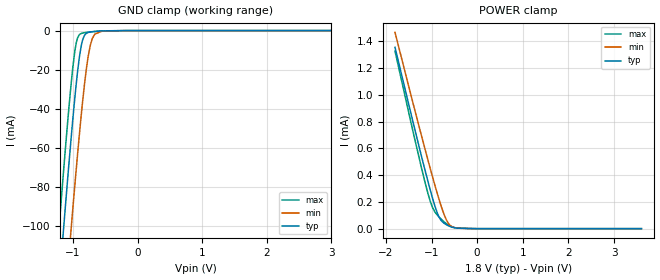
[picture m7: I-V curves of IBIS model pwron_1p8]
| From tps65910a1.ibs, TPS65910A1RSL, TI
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|   pwron_1p8 Model
[Model]   pwron_1p8
Model_type   Input
Vinl = 0.54
Vinh = 1.26
|   typ   min   max
|   (nom PVT)   (fast PVT)   (slow PVT)
C_comp   1.767e-13   1.755e-13   1.788e-13
[Model spec]
|subparameter
Vinl   0.54   0.495   0.585
Vinh   1.26   1.155   1.365
| Where nom  PVT is Nominal Process, 1.8V, 27C
|   Fast PVT is Strong Process,  1.95V, -40C
|   Slow PVT is Weak Process,   1.65V, 125C
[Voltage Range]   1.8   1.65   1.95
|Junction Temperature
[Temperature Range]   27   125   -40
[Power Clamp Reference]   1.8   1.65   1.95
[GND Clamp Reference]   0   0   0
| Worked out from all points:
|   GND clamp passes 1 mA (typ) near -0.77 V on its own axis
[GND Clamp]
|   Voltage   I(typ)   I(min)   I(max)
-1.8V     -386.3mA   -432.6mA   -358.2mA
-1.404V   -211.1mA   -258.7mA   -181.7mA
-1.205V   -125.8mA   -173.7mA   -96.01mA
-1.168V   -110.4mA   -158.2mA   -80.59mA
-1.123V   -91.91mA   -139.6mA   -62.35mA
-1.018V   -50.62mA   -96.93mA   -23.29mA
-948.6mV  -26.62mA   -70.23mA   -6.002mA
-876.6mV  -8.368mA   -44.47mA   -1.52mA
-803.4mV  -1.665mA   -22.12mA   -996.5uA
-733.3mV  -734.1uA   -7.619mA   -701.3uA
-551mV    -175.5uA   -315.4uA   -135.6uA
3.6V      0A         0A         0A
[POWER Clamp]
|   Voltage   I(typ)   I(min)   I(max)
-1.8V     1.356mA    1.467mA    1.327mA
-1.459V   872uA      1.009mA    806.4uA
-1.223V   545.7uA    698.7uA    458.8uA
-1.079V   354.4uA    514uA      264uA
-1.028V   289.3uA    449.6uA    204.8uA
-928.4mV  171.9uA    327.5uA    126.4uA
-817.2mV  75.48uA    199.3uA    81.15uA
-709.2mV  37.02uA    92.62uA    46.64uA
-603.8mV  17.64uA    28.36uA    21.21uA
-464.4mV  4.645uA    5.41uA     5.855uA
-180mV    1.035uA    621.9nA    1.718uA
3.6V      0A         0A         0A
